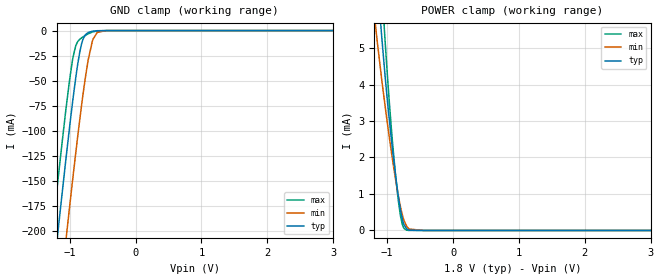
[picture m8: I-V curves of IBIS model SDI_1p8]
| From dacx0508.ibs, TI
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|   Model
[Model]   SDI_1p8
Model_type   Input
Vinl = 0.54
Vinh = 1.26
|   typ   min   max
C_comp   1.25791pF   1.11594pF   1.31717pF
| Where nom  PVT is Nominal Process, 1.8V, 27C
|   Fast PVT is Strong Process,  1.9V, -40C
|   Slow PVT is Weak Process,   1.7V, 125C
[Voltage Range]   1.8   1.7   1.9
|Junction Temperature
[Temperature Range]   27   125   -40
[Power Clamp Reference]   1.8   1.7   1.9
[GND Clamp Reference]   0   0   0
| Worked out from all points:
|   GND clamp passes 1 mA (typ) near -0.67 V on its own axis
|   POWER clamp passes 1 mA (typ) near -0.84 V on its own axis
[GND Clamp]
|   Voltage   I(typ)   I(min)   I(max)
-1.8V     -596.3mA   -677.4mA   -545.4mA
-1.211V   -221.2mA   -303.4mA   -169.5mA
-1.174V   -198mA     -280.1mA   -146.4mA
-1.06V    -129.9mA   -211mA     -80.03mA
-1.001V   -95.76mA   -175.6mA   -48.74mA
-963mV    -75mA      -153.5mA   -31.77mA
-909mV    -47.47mA   -122.6mA   -15.42mA
-822.6mV  -14.09mA   -76.04mA   -7.447mA
-720mV    -1.954mA   -29.5mA    -3.292mA
-644.4mV  -536.3uA   -8.355mA   -1.214mA
-444.6mV  -4.4uA     -43.35uA   -6.19uA
3.6V      0A         0A         0A
[POWER Clamp]
|   Voltage   I(typ)   I(min)   I(max)
-1.8V     23.89mA    18.22mA    29.42mA
-1.184V   7.681mA    5.73mA     9.698mA
-1.152V   6.898mA    5.193mA    8.709mA
-1.087V   5.401mA    4.196mA    6.774mA
-1.082V   5.282mA    4.117mA    6.616mA
-1.033V   4.257mA    3.428mA    5.231mA
-930.6mV  2.401mA    2.081mA    2.66mA
-828mV    898.3uA    920.7uA    776.1uA
-768.6mV  301.4uA    419.5uA    155.3uA
-703.8mV  42.07uA    113.7uA    8.686uA
-444.6mV  0A         67.7nA     0A
3.6V      0A         0A         0A
